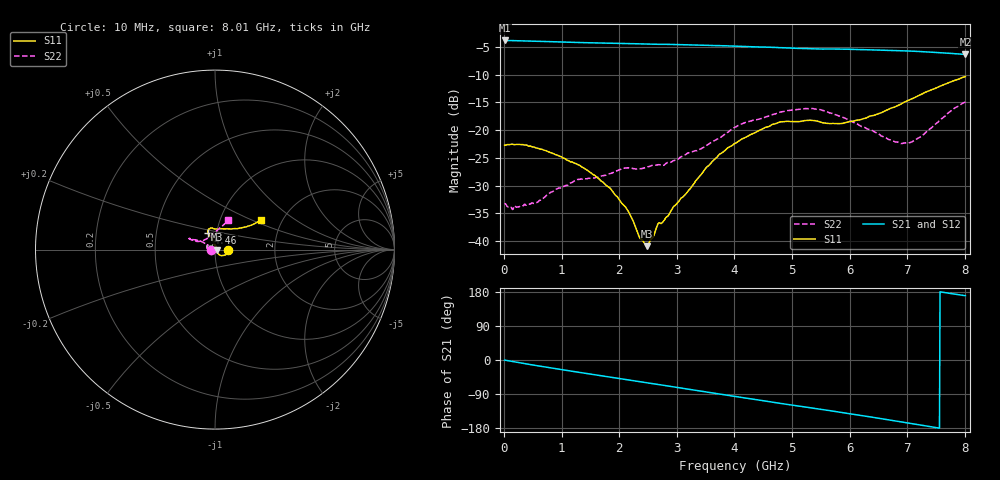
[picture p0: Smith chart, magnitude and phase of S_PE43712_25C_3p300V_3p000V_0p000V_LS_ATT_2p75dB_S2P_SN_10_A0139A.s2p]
! DEVICE ID: PE43712
! File Path: z:\PE43713\PE43713_CHAR_NOM_04292014\AMB\3p300\LS_ATT_2p75dB\PE43713_AMB_3p300V_3p000V_0p000V_LS_ATT_2p75dB_S2P_SN_10_A0139A.s2p
! Serial: 10
! Lot: A0139A
! Temp: 25C
! VDD: 3.300
! VSS: 0.000
! Control_Hi: 3.000
! Control_Lo: 0.000
! Attenuation Step: 2.75dB
! Port 1: RF1
! Port 2: RF2
! ThroughPath:1-2
! IDD: 0.0001468006
! ISS: -2.24e-008
#  Hz  S  RI  R  50
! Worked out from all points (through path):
!   801 points, 10 MHz to 8.01 GHz, reference 50 ohm
!   highest |S21| = -3.80 dB at 10 MHz (marker M1); lowest = -6.3 dB at 8.01 GHz (marker M2)
!   group delay of S21, straight-line fit = 65.2 ps
!   lowest |S11| = -40.9 dB at 2.48 GHz (marker M3), VSWR 1.02, Z = 50.9 - j0.076 ohm
!   |S11| at or under -10 dB: start of sweep to end of sweep
!   |S22| runs from -34.3 to -14.9 dB; largest |S21 - S12| = 0.0019
!   S11 on the Smith chart (normalised r, x): 10 MHz: 1.16, -0.00; 4.46 GHz: 0.91, +0.17; 8.01 GHz: 1.57, +0.56
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1e7  0.0734 -0.000445  0.6455 -0.00352  0.6454 -0.00359  -0.0217 -7.61e-05
1.3e8  0.0745 -0.00577  0.6427 -0.04  0.6425 -0.0399  -0.02 -0.000925
5.5e8  0.0647 -0.0248  0.6153 -0.1581  0.6149 -0.1582  -0.0207 -0.00822
9.1e8  0.0505 -0.032  0.5759 -0.2478  0.5759 -0.2478  -0.0274 -0.0106
1.35e9  0.0327 -0.0331  0.5138 -0.3424  0.5137 -0.3423  -0.0348 -0.00999
1.86e9  0.0181 -0.0229  0.4263 -0.4349  0.4262 -0.4348  -0.0408 -0.00102
2.14e9  0.0109 -0.0156  0.3713 -0.4778  0.3713 -0.4775  -0.0455 0.0044
2.35e9  0.00881 -0.00625  0.3268 -0.5054  0.3269 -0.5053  -0.0438 0.0103
2.48e9  0.00895 -0.000747  0.2983 -0.52  0.2983 -0.52  -0.0436 0.0166
2.58e9  0.00948 0.00521  0.276 -0.5293  0.2762 -0.5296  -0.043 0.0221
2.68e9  0.00989 0.0105  0.2548 -0.5387  0.255 -0.5387  -0.0405 0.0274
2.77e9  0.00876 0.0123  0.2348 -0.5477  0.2349 -0.5478  -0.0406 0.0261
3.51e9  -0.00909 0.045  0.058 -0.5803  0.0578 -0.5805  -0.0621 0.0375
4.01e9  -0.0244 0.0719  -0.0613 -0.5708  -0.061 -0.5708  -0.0932 0.0511
4.46e9  -0.0399 0.093  -0.1598 -0.5404  -0.1598 -0.5407  -0.1149 0.0542
4.8e9  -0.0371 0.113  -0.2303 -0.506  -0.2299 -0.5062  -0.1332 0.0589
5.35e9  -0.021 0.1207  -0.3254 -0.435  -0.3253 -0.4346  -0.1447 0.061
5.86e9  0.0134 0.1138  -0.4035 -0.3578  -0.4026 -0.3579  -0.1208 0.052
6.68e9  0.1024 0.1159  -0.4867 -0.1962  -0.4864 -0.1959  -0.0645 0.0509
6.9e9  0.128 0.1168  -0.4993 -0.1484  -0.499 -0.1483  -0.0457 0.0605
7.1e9  0.1507 0.1219  -0.506 -0.1037  -0.5054 -0.1036  -0.026 0.0751
8.01e9  0.2578 0.1627  -0.475 0.0856  -0.4737 0.0847  0.0737 0.1636
